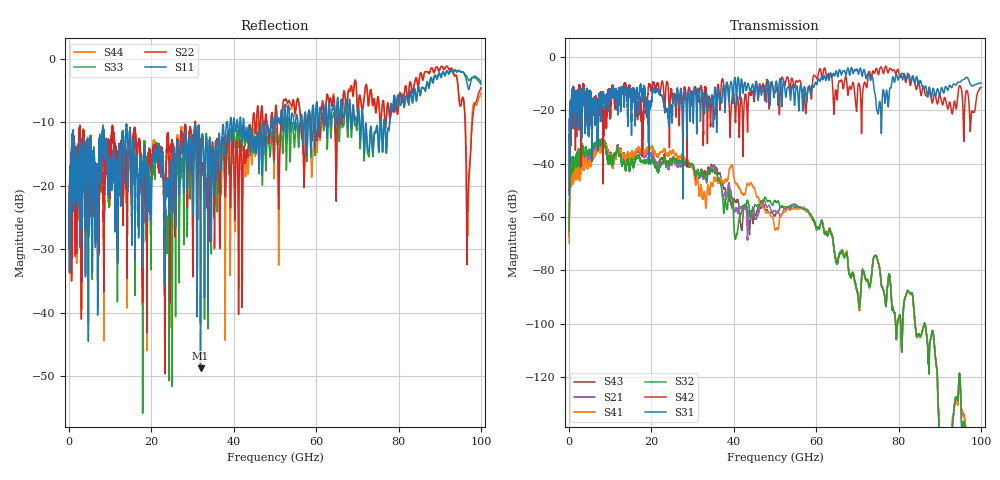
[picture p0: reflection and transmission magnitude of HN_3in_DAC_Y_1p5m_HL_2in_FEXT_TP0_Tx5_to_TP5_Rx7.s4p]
# GHz S RI R 45
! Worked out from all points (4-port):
!   4000 points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, 25 MHz to 100 GHz, reference 45 ohm
!   strongest paths, dB at 25 MHz, 25.02 GHz, 50.02 GHz, 75.03 GHz, 100 GHz:
!     S31: -51.8, -23.3, -11.7, -21.4, -9.9
!     S42: -50.1, -13.8, -13.1, -6.4, -11.5
!     S32: -65.3, -39.2, -53.9, -76.8, -183.0
!     S41: -69.8, -36.0, -64.7, -76.7, -183.6
!     S21: -67.5, -40.1, -57.8, -76.7, -181.0
!     S43: -67.3, -38.7, -59.4, -76.7, -184.8
!   lowest |S11| = -48.8 dB at 31.93 GHz (marker M1), VSWR 1.01, Z = 45.3 + j0.168 ohm
!   |S11| at or under -10 dB: start of sweep to 38.27 GHz; 42.47 GHz to 47.28 GHz (4.815 GHz wide, 10.7 % of centre); 71.39 GHz to 75.58 GHz (4.195 GHz wide, 5.71 % of centre)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
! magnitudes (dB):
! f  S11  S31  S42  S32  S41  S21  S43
! 25 MHz  -24.7  -51.8  -50.1  -65.3  -69.8  -67.5  -67.3
! 1.2 GHz  -24.0  -26.9  -16.2  -40.3  -44.5  -42.5  -42.7
! 8.35 GHz  -11.2  -13.3  -33.3  -32.5  -33.3  -32.7  -32.4
! 31.93 GHz  -48.8  -23.7  -11.7  -43.5  -48.6  -44.8  -43.4
! 40.55 GHz  -11.3  -13.0  -20.3  -67.6  -47.4  -56.7  -54.3
! 68.38 GHz  -8.7  -5.0  -11.9  -82.4  -82.4  -82.2  -82.6
! 100 GHz  -3.6  -9.9  -11.5  -183.0  -183.6  -181.0  -184.8
